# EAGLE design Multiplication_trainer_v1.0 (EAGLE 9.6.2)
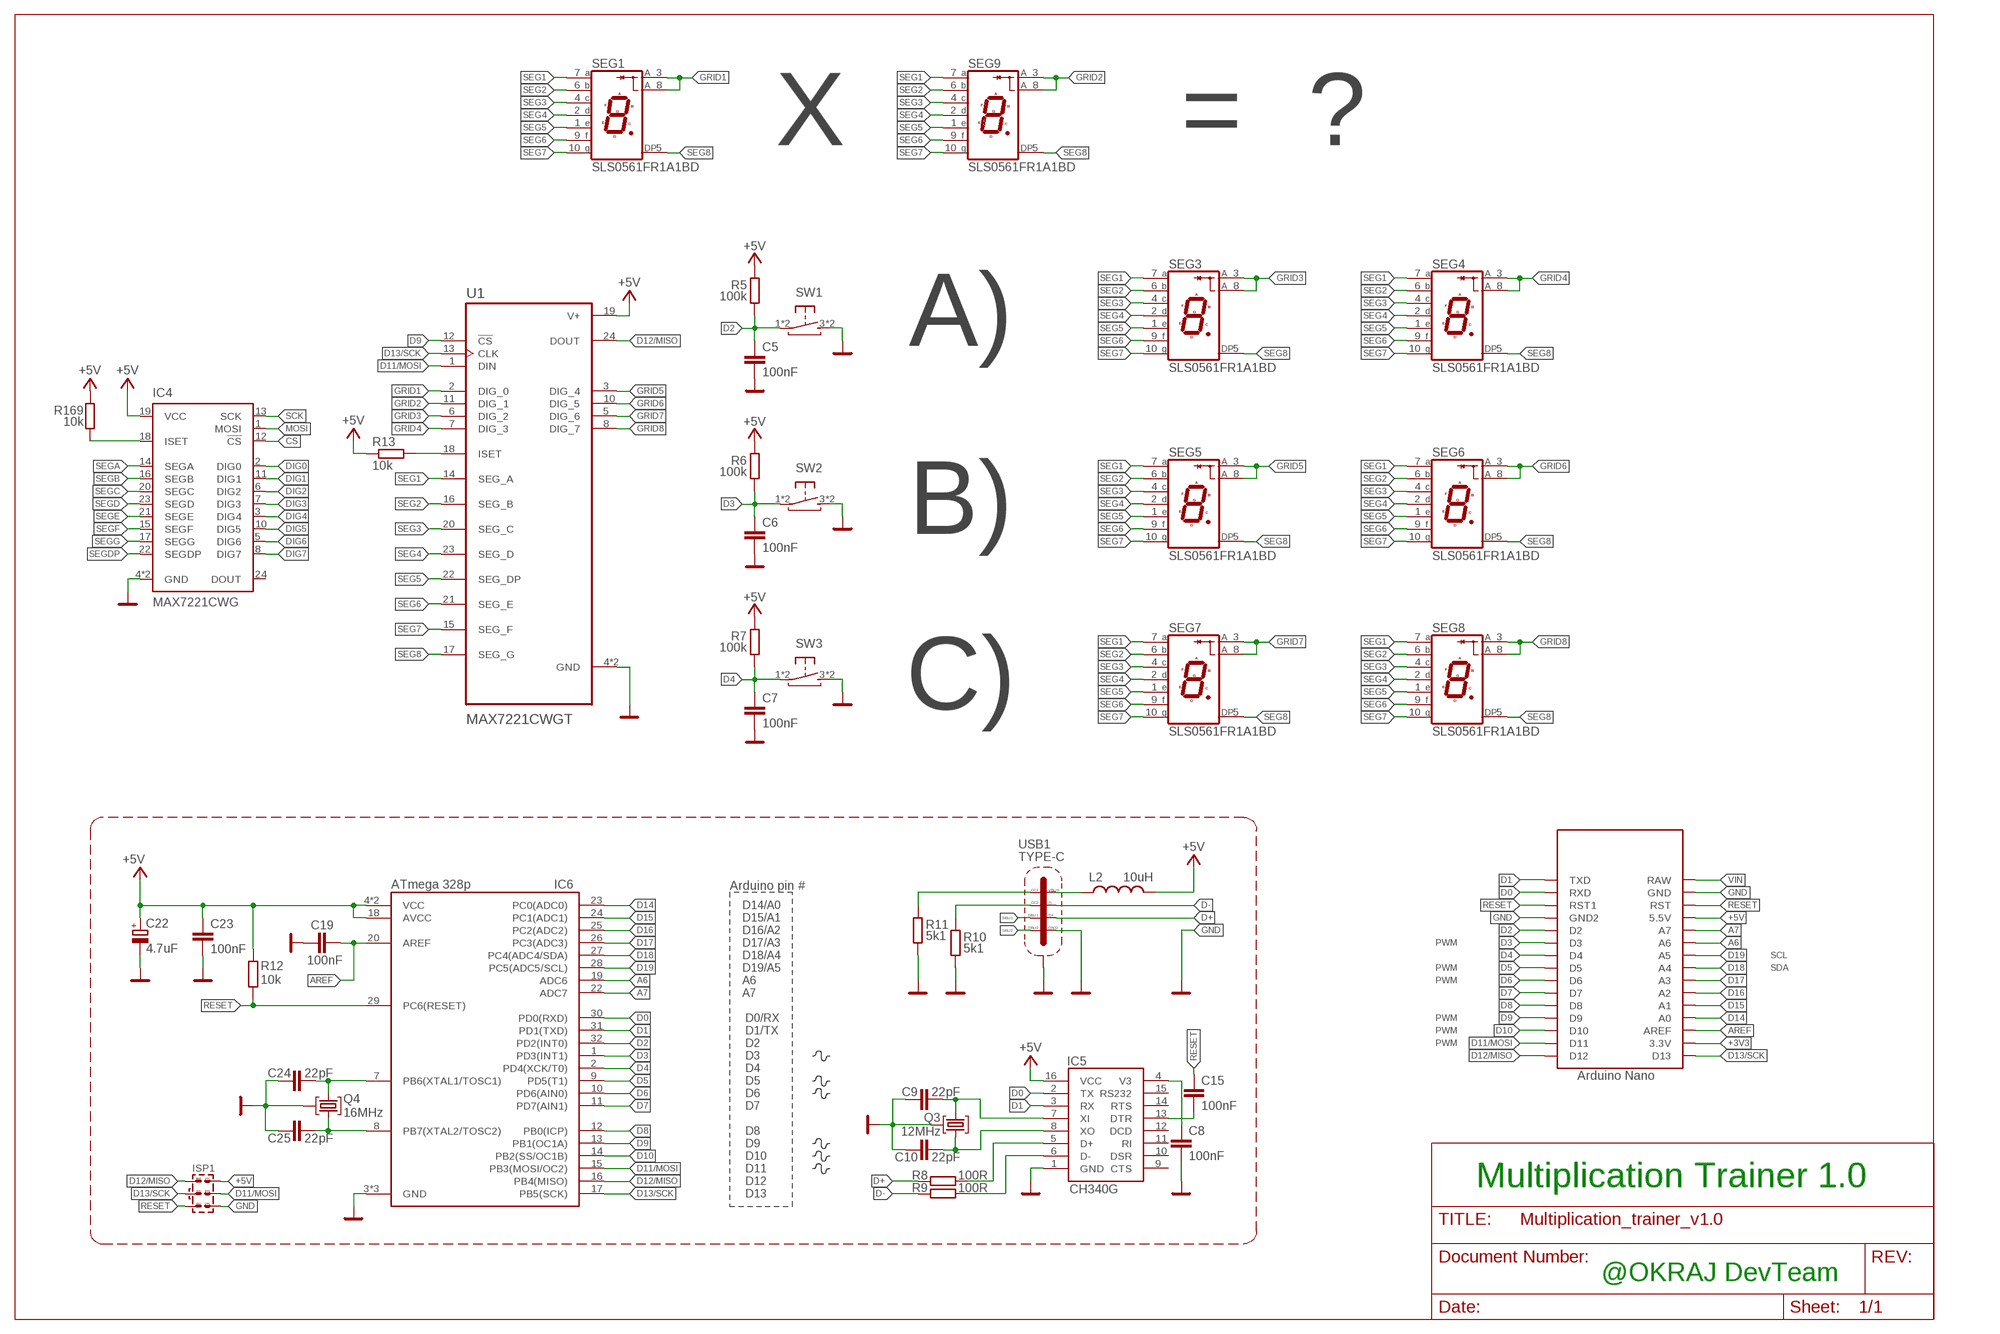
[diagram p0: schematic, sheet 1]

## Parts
C5  100nF  C-EUC0805  [C0805]
C6  100nF  C-EUC0805  [C0805]
C7  100nF  C-EUC0805  [C0805]
C8  100nF  C-EUC0603  [C0603]
C9  22pF  C-EUC0603  [C0603]
C10  22pF  C-EUC0603  [C0603]
C15  100nF  C-EUC0603  [C0603]
C19  100nF  C-EUC0603  [C0603]
C22  4.7uF  CPOL-EUSMCA  [SMC_A]
C23  100nF  C-EUC0603  [C0603]
C24  22pF  C-EUC0603  [C0603]
C25  22pF  C-EUC0603  [C0603]
IC4  MAX7221CWG  [SOIC127P1032X265-24N]
IC5  CH340G  CH340GSMD  [SOIC16]
IC6  ATmega 328p  ATMEGA328PQFP32N_ROUND-PADS  [QFP80P900X900X120-32N_ROUND-PADS]
ISP1  AVR-ISP-SPI  [AVR-ISP-SPI]
L2  10uH  L-USL0805  [R0805]
Q3  12MHz  KRYSTAL  [ILCX13-FF5F18-16.0000]
Q4  16MHz  KRYSTAL  [ILCX13-FF5F18-16.0000]
R5  100k  R-EU_R0805  [R0805]
R6  100k  R-EU_R0805  [R0805]
R7  100k  R-EU_R0805  [R0805]
R8  100R  R-EU_R0603  [R0603]
R9  100R  R-EU_R0603  [R0603]
R10  5k1  R-EU_R0603  [R0603]
R11  5k1  R-EU_R0603  [R0603]
R12  10k  R-EU_R0603  [R0603]
R13  10k  R-EU_R0805  [R0805]
R169  10k  R-EU_R0805  [R0805]
SEG1  SLS0561FR1A1BD  [SLS0561FR1A1BD]
SEG3  SLS0561FR1A1BD  [SLS0561FR1A1BD]
SEG4  SLS0561FR1A1BD  [SLS0561FR1A1BD]
SEG5  SLS0561FR1A1BD  [SLS0561FR1A1BD]
SEG6  SLS0561FR1A1BD  [SLS0561FR1A1BD]
SEG7  SLS0561FR1A1BD  [SLS0561FR1A1BD]
SEG8  SLS0561FR1A1BD  [SLS0561FR1A1BD]
SEG9  SLS0561FR1A1BD  [SLS0561FR1A1BD]
SW1  TACT-SW_BTNSMTJLC_6X6X4.5  [TACTSW_6X6X4.5_SMT]
SW2  TACT-SW_BTNSMTJLC_6X6X4.5  [TACTSW_6X6X4.5_SMT]
SW3  TACT-SW_BTNSMTJLC_6X6X4.5  [TACTSW_6X6X4.5_SMT]
U1  MAX7221CWGT  [SOIC127P1032X265-24N]
U$2  NANOTHT-NOUSB  [NANO-NOUSB]
USB1  TYPE-C  TYPE-C-31-M-12TYPE-C-31_L8.94_W7.3  [TYPE-C-31_L8.94_W7.3]

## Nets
+3V3: U$2.3.3V
+5V: C22.+ C23.1 IC4.19(VCC) IC5.16(VCC) IC6.4(VCC) IC6.6(VCC) IC6.18(AVCC) ISP1.2 L2.2 R5.1 R6.1 R7.1 R12.1 R13.1 R169.2 U1.19(V+) U$2.5V(5.5V)
A6: IC6.19(ADC6) U$2.A6
A7: IC6.22(ADC7) U$2.A7
AREF: C19.1 IC6.20(AREF) U$2.AREF
CS: IC4.12(!CS)
D0: IC5.2(TX) IC6.30(PD0(RXD)) U$2.RX1(RXD)
D1: IC5.3(RX) IC6.31(PD1(TXD)) U$2.TX0(TXD)
D2: C5.1 IC6.32(PD2(INT0)) R5.2 SW1.1(P) SW1.2(P) U$2.D2
D3: C6.1 IC6.1(PD3(INT1)) R6.2 SW2.1(P) SW2.2(P) U$2.D3
D4: C7.1 IC6.2(PD4(XCK/T0)) R7.2 SW3.1(P) SW3.2(P) U$2.D4
D5: IC6.9(PD5(T1)) U$2.D5
D6: IC6.10(PD6(AIN0)) U$2.D6
D7: IC6.11(PD7(AIN1)) U$2.D7
D8: IC6.12(PB0(ICP)) U$2.D8
D9: IC6.13(PB1(OC1A)) U1.12(!CS) U$2.D9
D10: IC6.14(PB2(SS/OC1B)) U$2.D10
D11/MOSI: IC6.15(PB3(MOSI/OC2)) ISP1.4 U1.1(DIN) U$2.D11
D12/MISO: IC6.16(PB4(MISO)) ISP1.1 U1.24(DOUT) U$2.D12
D13/SCK: IC6.17(PB5(SCK)) ISP1.3 U1.13(CLK) U$2.D13
D14: IC6.23(PC0(ADC0)) U$2.A0
D15: IC6.24(PC1(ADC1)) U$2.A1
D16: IC6.25(PC2(ADC2)) U$2.A2
D17: IC6.26(PC3(ADC3)) U$2.A3
D18: IC6.27(PC4(ADC4/SDA)) U$2.A4
D19: IC6.28(PC5(ADC5/SCL)) U$2.A5
D+: R8.1 USB1.A6(D+) USB1.B6(D+)
D-: R9.1 USB1.A7(D-) USB1.B7(D-)
DIG0: IC4.2(DIG0)
DIG1: IC4.11(DIG1)
DIG2: IC4.6(DIG2)
DIG3: IC4.7(DIG3)
DIG4: IC4.3(DIG4)
DIG5: IC4.10(DIG5)
DIG6: IC4.5(DIG6)
DIG7: IC4.8(DIG7)
GND: C5.2 C6.2 C7.2 C8.2 C9.2 C10.2 C19.2 C22.- C23.2 C24.2 C25.2 IC4.4(GND) IC4.9(GND) IC5.1(GND) IC6.3(GND) IC6.5(GND) IC6.21(GND) ISP1.6 Q3.P$2(GND) Q3.P$4(GND) Q4.P$2(GND) Q4.P$4(GND) R10.1 R11.1 SW1.3(S) SW1.4(S) SW2.3(S) SW2.4(S) SW3.3(S) SW3.4(S) U1.4(GND) U1.9(GND) U$2.GND U$2.GND1(GND2) USB1.A1/B12(GND) USB1.B1/A12(GND) USB1.SHIELD1(SHIELD) USB1.SHIELD2(SHIELD) USB1.SHIELD3(SHIELD) USB1.SHIELD4(SHIELD) USB1.SHIELD5(SHIELD) USB1.SHIELD6(SHIELD) USB1.SHIELD7(SHIELD) USB1.SHIELD8(SHIELD)
GRID1: SEG1.3(CA1) SEG1.8(CA2) U1.2(DIG_0)
GRID2: SEG9.3(CA1) SEG9.8(CA2) U1.11(DIG_1)
GRID3: SEG3.3(CA1) SEG3.8(CA2) U1.6(DIG_2)
GRID4: SEG4.3(CA1) SEG4.8(CA2) U1.7(DIG_3)
GRID5: SEG5.3(CA1) SEG5.8(CA2) U1.3(DIG_4)
GRID6: SEG6.3(CA1) SEG6.8(CA2) U1.10(DIG_5)
GRID7: SEG7.3(CA1) SEG7.8(CA2) U1.5(DIG_6)
GRID8: SEG8.3(CA1) SEG8.8(CA2) U1.8(DIG_7)
MOSI: IC4.1(MOSI)
N$1: C8.1 IC5.4(V3)
N$2: C9.1 IC5.7(XI) Q3.P$1
N$3: C10.1 IC5.8(XO) Q3.P$3
N$4: C15.2 IC5.13(DTR)
N$5: IC5.5(D+) R8.2
N$8: IC5.6(D-) R9.2
N$9: L2.1 USB1.A4/B9(VBUS) USB1.B4/A9(VBUS)
N$10: R10.2 USB1.B5(CC2)
N$11: R11.2 USB1.A5(CC1)
N$12: C24.1 IC6.7(PB6(XTAL1/TOSC1)) Q4.P$1
N$13: C25.1 IC6.8(PB7(XTAL2/TOSC2)) Q4.P$3
N$14: R13.2 U1.18(ISET)
N$131: IC4.18(ISET) R169.1
RESET: C15.1 IC6.29(PC6(RESET)) ISP1.5 R12.2 U$2.RST U$2.RST1
SBU1: USB1.A8(SBU1)
SBU2: USB1.B8(SBU2)
SCK: IC4.13(SCK)
SEG1: SEG1.7(A) SEG3.7(A) SEG4.7(A) SEG5.7(A) SEG6.7(A) SEG7.7(A) SEG8.7(A) SEG9.7(A) U1.14(SEG_A)
SEG2: SEG1.6(B) SEG3.6(B) SEG4.6(B) SEG5.6(B) SEG6.6(B) SEG7.6(B) SEG8.6(B) SEG9.6(B) U1.16(SEG_B)
SEG3: SEG1.4(C) SEG3.4(C) SEG4.4(C) SEG5.4(C) SEG6.4(C) SEG7.4(C) SEG8.4(C) SEG9.4(C) U1.20(SEG_C)
SEG4: SEG1.2(D) SEG3.2(D) SEG4.2(D) SEG5.2(D) SEG6.2(D) SEG7.2(D) SEG8.2(D) SEG9.2(D) U1.23(SEG_D)
SEG5: SEG1.1(E) SEG3.1(E) SEG4.1(E) SEG5.1(E) SEG6.1(E) SEG7.1(E) SEG8.1(E) SEG9.1(E) U1.22(SEG_DP)
SEG6: SEG1.9(F) SEG3.9(F) SEG4.9(F) SEG5.9(F) SEG6.9(F) SEG7.9(F) SEG8.9(F) SEG9.9(F) U1.21(SEG_E)
SEG7: SEG1.10(G) SEG3.10(G) SEG4.10(G) SEG5.10(G) SEG6.10(G) SEG7.10(G) SEG8.10(G) SEG9.10(G) U1.15(SEG_F)
SEG8: SEG1.5(DP) SEG3.5(DP) SEG4.5(DP) SEG5.5(DP) SEG6.5(DP) SEG7.5(DP) SEG8.5(DP) SEG9.5(DP) U1.17(SEG_G)
SEGA: IC4.14(SEGA)
SEGB: IC4.16(SEGB)
SEGC: IC4.20(SEGC)
SEGD: IC4.23(SEGD)
SEGDP: IC4.22(SEGDP)
SEGE: IC4.21(SEGE)
SEGF: IC4.15(SEGF)
SEGG: IC4.17(SEGG)
VIN: U$2.RAW
Unconnected: IC4.24(DOUT) IC5.9(CTS) IC5.10(DSR) IC5.11(RI) IC5.12(DCD) IC5.14(RTS) IC5.15(RS232)

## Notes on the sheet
- X | = | ?
- A)
- B)
- C)
- Arduino pin #
- D14/A0
- D15/A1
- D16/A2
- D17/A3 | PWM
- D18/A4 | SCL
- D19/A5 | PWM | SDA
- A6 | PWM
- A7
- D0/RX | PWM
- D1/TX | PWM
- D2 | PWM
- D3
- D4
- D5
- D6
- D7
- D8
- D9
- D10
- D11
- D12
- Multiplication Trainer 1.0
- D13
- @OKRAJ DevTeam

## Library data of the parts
C5-C7 = rcl:C-EU: CAPACITOR, European symbol
C8 C15 C19 C23 = rcl:C-EU: CAPACITOR, European symbol; LCSC_PART: C49678; SPICEPREFIX: C
C9 C10 C24 C25 = rcl:C-EU: CAPACITOR, European symbol; LCSC_PART: C1804; SPICEPREFIX: C
C22 = rcl:CPOL-EU: POLARIZED CAPACITOR, European symbol; LCSC_PART: C111040; ROT: 180; SPICEPREFIX: C
IC4 = MAX7221:MAX7221CWG: 7 SEGMENT 8 DIGIT DRIVER 24SOIC Datasheet; MOUSER_NO: 710-157119S12701
IC5 = ch340g:CH340G; LCSC_PART: C14267
IC6 = ATMEGA328P-ANR:ATMEGA328P: 8-bit Microcontrollers - MCU AVR 32K FLSH 2K SRAM 1KB EE-20 MHZ 105C Source: Datasheet; LCSC_PART: C14877; ROT: 270
ISP1 = #Ondra2:AVR-ISP-SPI
L2 = rcl:L-US: INDUCTOR, American symbol; LCSC_PART: C281113
Q3 = #Marek:KRYSTAL: Monolithic Crystal Filters Source: www.vanlong.com; LCSC_PART: C9002
Q4 = #Marek:KRYSTAL: Monolithic Crystal Filters Source: www.vanlong.com; LCSC_PART: C13738
R5-R7 = resistor:R-EU_: RESISTOR, European symbol
R8 R9 R12 R13 R169 = rcl:R-EU_: RESISTOR, European symbol; SPICEPREFIX: R
R10 R11 = rcl:R-EU_: RESISTOR, European symbol; LCSC_PART: C27834; SPICEPREFIX: R
SEG1 SEG3-SEG9 = #my:SLS0561FR1A1BD; LCSC_PART: C226002
SW1-SW3 = #Ondra2:TACT-SW_BTN; LCSC_PART: C127509
U1 = MAX7221CWGT:MAX7221CWGT: Check availability; AVAILABILITY: In Stock; DESCRIPTION: IC DRVR 7 SEGMNT 8 DIGIT 24SOIC; MF: Maxim Integrated; MP: MAX7221CWG+T; PACKAGE: SOIC-24 Maxim; PRICE: None; PURCHASE-URL: https://pricing.snapeda.com/search/part/MAX7221CWG+T/?ref=eda
U$2 = Arduino-clone:NANO: Arduino Nano
USB1 = #Marek:TYPE-C-31-M-12; LCSC_PART: C165948; ROT: 180

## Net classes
0 default: width 0.127 mm, drill 0.2 mm, clearance 0.127 mm

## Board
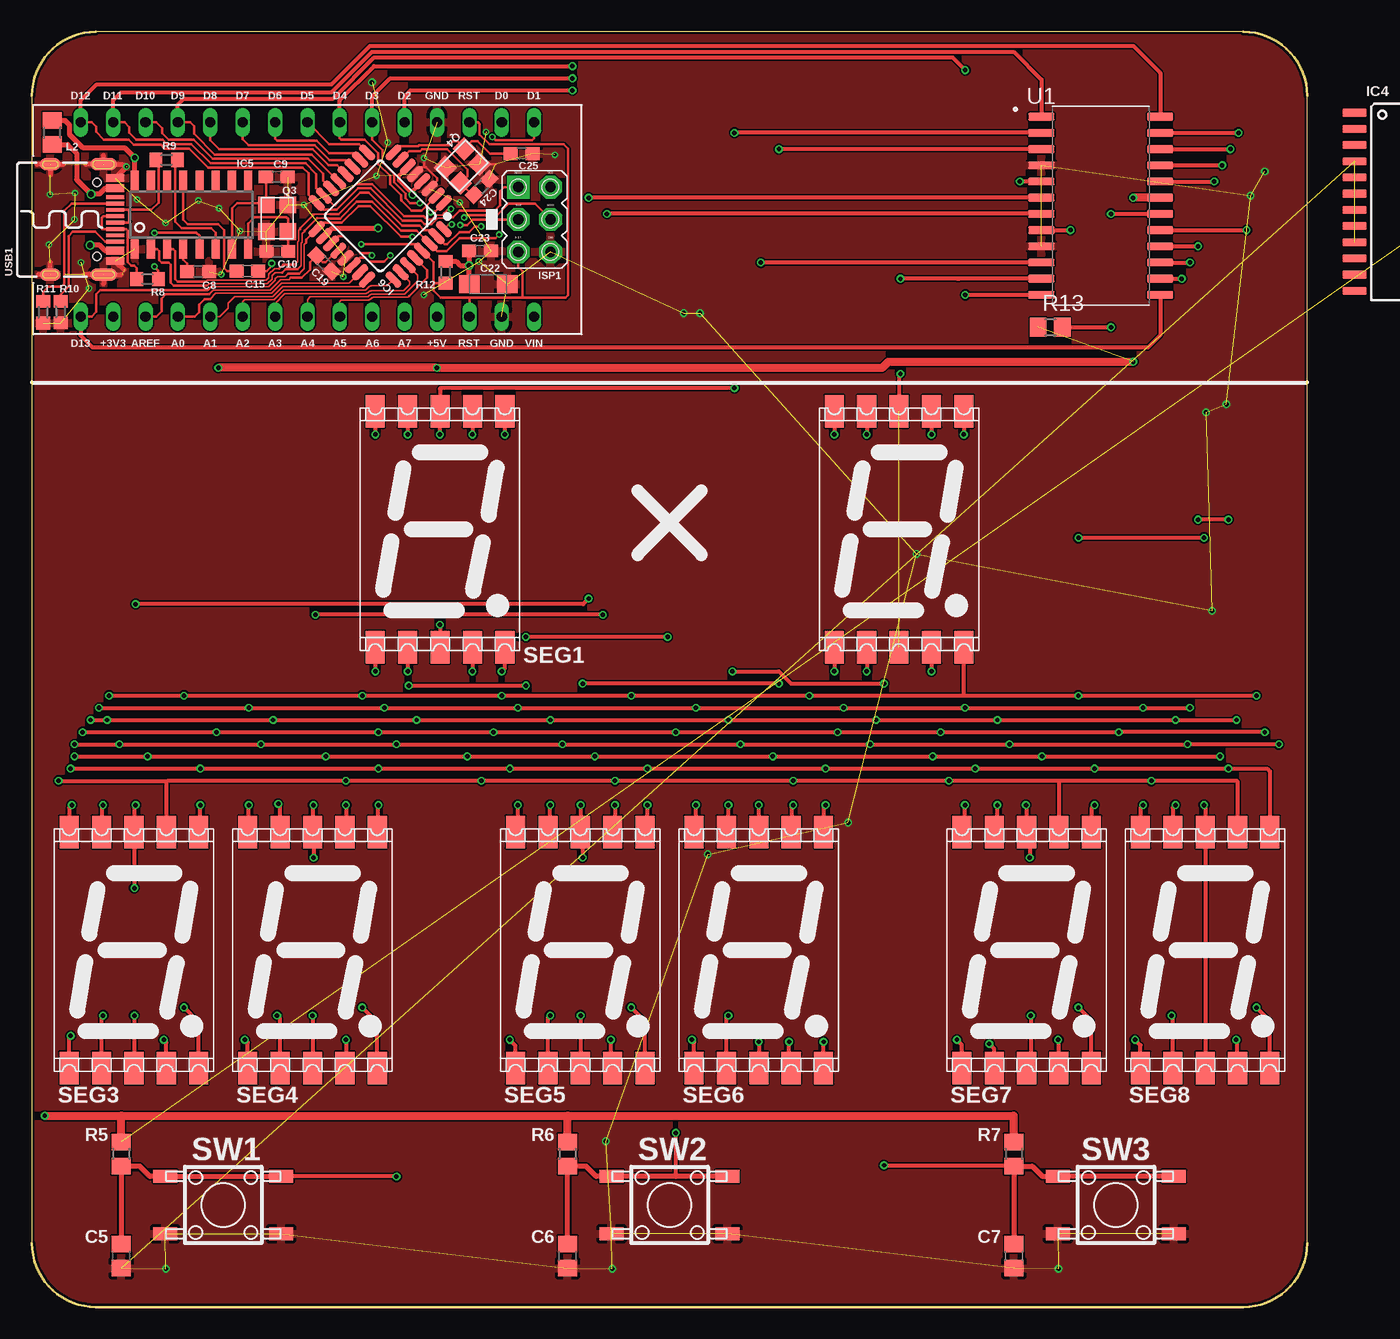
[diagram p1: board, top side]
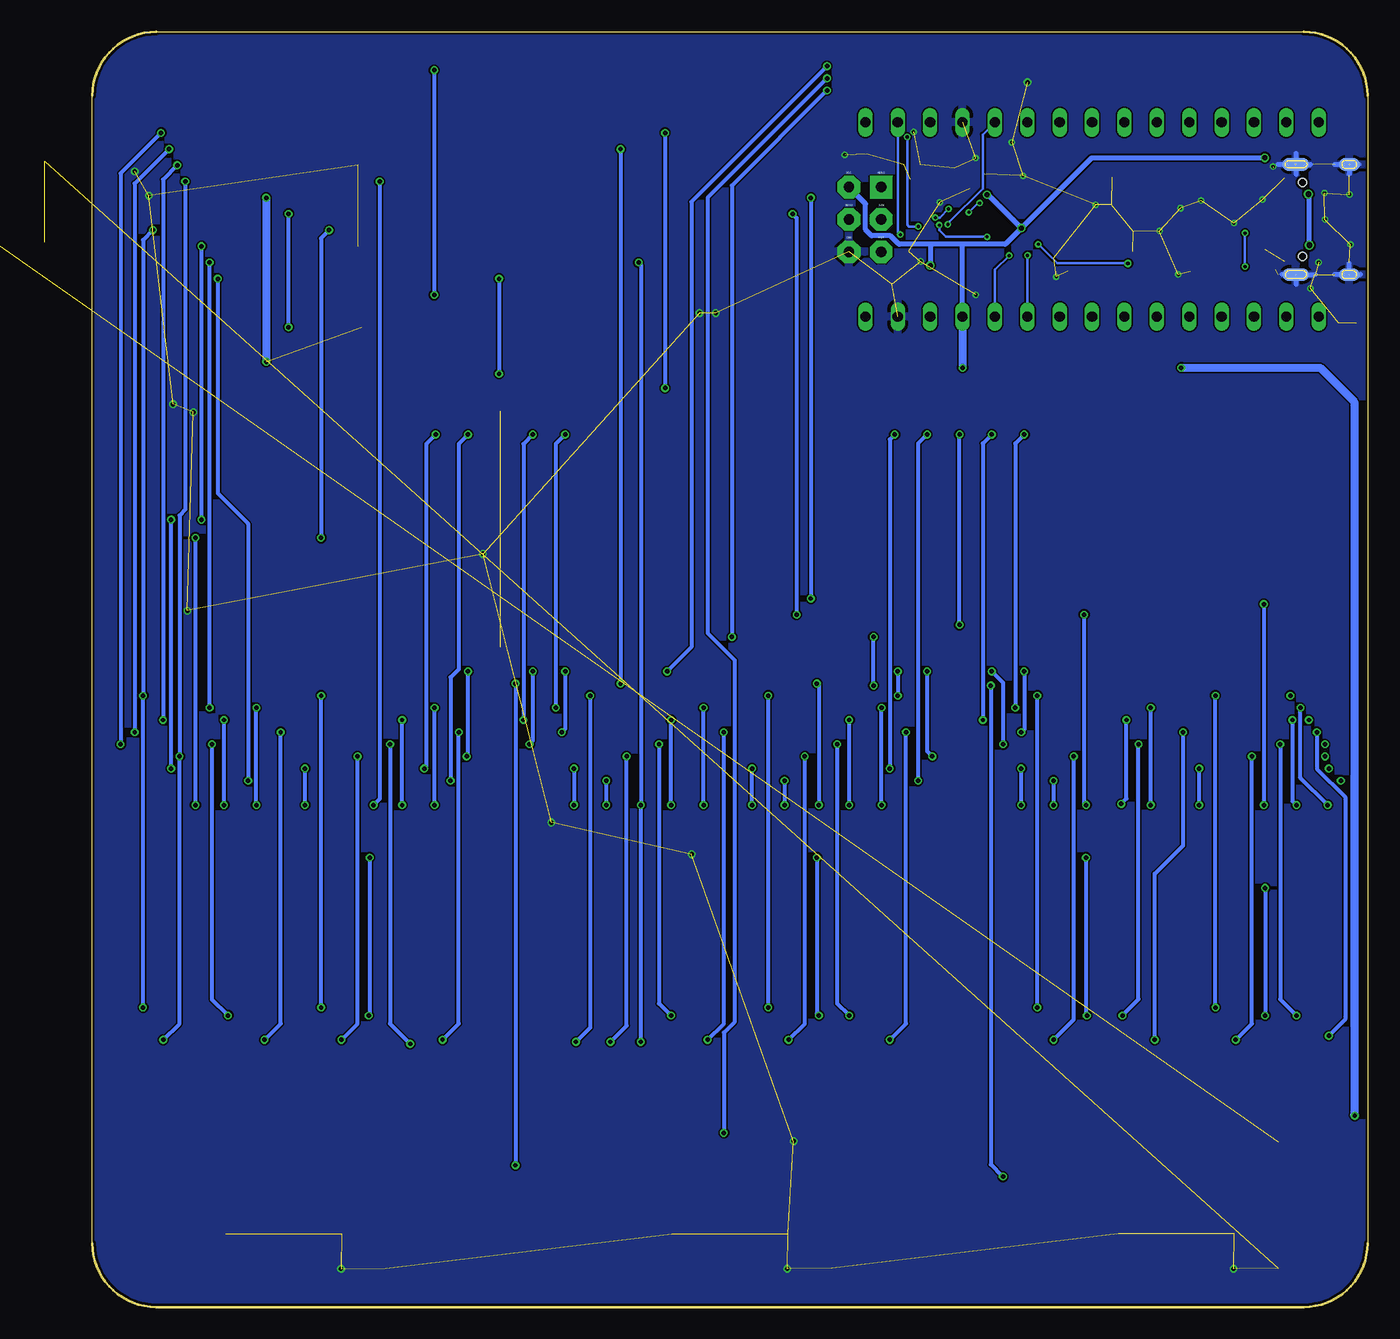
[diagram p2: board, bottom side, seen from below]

Size 100 x 100 mm. Coordinates in mm from the lower left corner, seen from the top.
Outline: 100,5 100,95 arc90 95,100 5,100 arc90 0,95 0,5 arc90 5,0 95,0 arc90 100,5
Copper layers (1*16): Top 0.035mm / dielectric 1.6mm / Bottom 0.035mm
Design rules "jlcpcb-2layers_od-Ondry3-assembly-tight": minimum track width 5mil, minimum drill 0.2mm, track to track 5mil, track to pad 5mil, pad to pad 5mil, via to via 5mil, smd to smd 5mil, copper to edge 0.2mm, drill to drill 6mil, minimum pad ring 0.13mm, minimum via ring 0.13mm, stop-mask expansion 4mil, vias tented up to drill 0.6mm, thermal gap 10mil

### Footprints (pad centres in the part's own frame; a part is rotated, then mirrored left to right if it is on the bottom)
C0805 = smd 1.3 x 1.5: 1 -0.95,0; 2 0.95,0
C0603 = smd 1.1 x 1: 1 -0.85,0; 2 0.85,0
SMC_A = smd 1.6 x 1.4: + -1.5,0; - 1.5,0
SOIC127P1032X265-24N = smd 1.925 x 0.65: 1 -4.712,6.985; 2 -4.712,5.715; 3 -4.712,4.445; 4 -4.712,3.175; 5 -4.712,1.905; 6 -4.712,0.635; 7 -4.712,-0.635; 8 -4.712,-1.905; 9 -4.712,-3.175; 10 -4.712,-4.445; 11 -4.712,-5.715; 12 -4.712,-6.985; 13 4.712,-6.985; 14 4.712,-5.715; 15 4.712,-4.445; 16 4.712,-3.175; 17 4.712,-1.905; 18 4.712,-0.635; 19 4.712,0.635; 20 4.712,1.905; 21 4.712,3.175; 22 4.712,4.445; 23 4.712,5.715; 24 4.712,6.985
SOIC16 = smd 0.635 x 1.524: 1 -4.445,-2.695; 2 -3.175,-2.695; 3 -1.905,-2.695; 4 -0.635,-2.695; 5 0.635,-2.695; 6 1.905,-2.695; 7 3.175,-2.695; 8 4.445,-2.695; 9 4.445,2.695; 10 3.175,2.695; 11 1.905,2.695; 12 0.635,2.695; 13 -0.635,2.695; 14 -1.905,2.695; 15 -3.175,2.695; 16 -4.445,2.695
QFP80P900X900X120-32N_ROUND-PADS = smd 1.499 x 0.584: 1 -4.25,2.8; 2 -4.25,2; 3 -4.25,1.2; 4 -4.25,0.4; 5 -4.25,-0.4; 6 -4.25,-1.2; 7 -4.25,-2; 8 -4.25,-2.8; 17 4.25,-2.8; 18 4.25,-2; 19 4.25,-1.2; 20 4.25,-0.4; 21 4.25,0.4; 22 4.25,1.2; 23 4.25,2; 24 4.25,2.8 | smd 0.584 x 1.499: 9 -2.8,-4.25; 10 -2,-4.25; 11 -1.2,-4.25; 12 -0.4,-4.25; 13 0.4,-4.25; 14 1.2,-4.25; 15 2,-4.25; 16 2.8,-4.25; 25 2.8,4.25; 26 2,4.25; 27 1.2,4.25; 28 0.4,4.25; 29 -0.4,4.25; 30 -1.2,4.25; 31 -2,4.25; 32 -2.8,4.25
AVR-ISP-SPI = drill 0.813 pad 1.778 square: 1 -1.27,2.54 | drill 0.813 pad 1.778 octagon: 2 1.27,2.54; 3 -1.27,0; 4 1.27,0; 5 -1.27,-2.54; 6 1.27,-2.54
R0805 = smd 1.3 x 1.5: 1 -0.95,0; 2 0.95,0
ILCX13-FF5F18-16.0000 = smd 1.3 x 1.3: P$1 -1.05,-0.85; P$2 1.05,-0.85; P$3 1.05,0.85; P$4 -1.05,0.85
R0603 = smd 1 x 1.1: 1 -0.85,0; 2 0.85,0
SLS0561FR1A1BD = smd 1.5 x 2.54: 1 -5.08,-9.25; 2 -2.54,-9.25; 3 0,-9.25; 4 2.54,-9.25; 5 5.08,-9.25; 6 5.08,9.25; 7 2.54,9.25; 8 0,9.25; 9 -2.54,9.25; 10 -5.08,9.25
TACTSW_6X6X4.5_SMT = smd 1.9 x 1: 1 -4.55,2.25; 2 4.55,2.25; 3 -4.55,-2.25; 4 4.55,-2.25
SOIC127P1032X265-24N' = smd 2.05 x 0.59: 1 -4.655,6.985; 2 -4.655,5.715; 3 -4.655,4.445; 4 -4.655,3.175; 5 -4.655,1.905; 6 -4.655,0.635; 7 -4.655,-0.635; 8 -4.655,-1.905; 9 -4.655,-3.175; 10 -4.655,-4.445; 11 -4.655,-5.715; 12 -4.655,-6.985; 13 4.655,-6.985; 14 4.655,-5.715; 15 4.655,-4.445; 16 4.655,-3.175; 17 4.655,-1.905; 18 4.655,-0.635; 19 4.655,0.635; 20 4.655,1.905; 21 4.655,3.175; 22 4.655,4.445; 23 4.655,5.715; 24 4.655,6.985
NANO-NOUSB = drill 0.8 long: 3.3V -7.62,15.24; 5V -7.62,-10.16; A0 -7.62,10.16; A1 -7.62,7.62; A2 -7.62,5.08; A3 -7.62,2.54; A4 -7.62,0; A5 -7.62,-2.54; A6 -7.62,-5.08; A7 -7.62,-7.62; AREF -7.62,12.7; D2 7.62,-7.62; D3 7.62,-5.08; D4 7.62,-2.54; D5 7.62,0; D6 7.62,2.54; D7 7.62,5.08; D8 7.62,7.62; D9 7.62,10.16; D10 7.62,12.7; D11 7.62,15.24; D12 7.62,17.78; D13 -7.62,17.78; GND -7.62,-15.24; GND1 7.62,-10.16; RAW -7.62,-17.78; RST -7.62,-12.7; RST1 7.62,-12.7; RX1 7.62,-15.24; TX0 7.62,-17.78
TYPE-C-31_L8.94_W7.3 = smd 0.6 x 1.45: A1/B12 -3.25,3.885; A4/B9 -2.45,3.885; B1/A12 3.25,3.885; B4/A9 2.45,3.885 | smd 0.3 x 1.45: A5 -1.25,3.885; A6 -0.25,3.885; A7 0.25,3.885; A8 1.25,3.885; B5 1.75,3.885; B6 0.75,3.885; B7 -0.75,3.885; B8 -1.75,3.885 | smd 1 x 2.1: SHIELD1 -4.32,2.97; SHIELD2 4.32,2.97 | smd 1 x 1.6: SHIELD3 -4.32,-1.21; SHIELD4 4.32,-1.21 | smd 1 x 2.1 bottom: SHIELD5 -4.316,2.97; SHIELD8 4.316,2.97 | smd 1 x 1.6 bottom: SHIELD6 -4.316,-1.21; SHIELD7 4.316,-1.21 | hole 0.65: -2.89,2.44; 2.89,2.44

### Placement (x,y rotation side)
C5  7,4 270 top
C6  42,4 270 top
C7  77,4 270 top
C8  13.04,81.2 0 top
C9  19.19,88.62 0 top
C10  19.25,82.78 180 top
C15  16.89,81.24 180 top
C19  22.91,81.85 315 top
C22  35.79,80.23 0 top
C23  35.14,82.82 0 top
C24  35.26,87.83 45 top
C25  38.39,90.46 0 top
IC4  not placed on the board
IC5  12.51,85.66 0 top
IC6  27.31,85.56 225 top
ISP1  39.4,85.29 0 top
L2  1.59,92.11 90 top
Q3  19.22,85.38 270 top
Q4  33.75,89.49 45 top
R5  7,12 270 top
R6  42,12 270 top
R7  77,12 270 top
R8  9.06,80.62 0 top
R9  10.56,89.96 0 top
R10  2.24,78.02 90 top
R11  0.87,78.02 90 top
R12  32.44,81.15 270 top
R13  79.85,76.83 0 top
R169  not placed on the board
SEG1  32,61 0 top
SEG3  8,28 0 top
SEG4  22,28 0 top
SEG5  43,28 0 top
SEG6  57,28 0 top
SEG7  78,28 0 top
SEG8  92,28 0 top
SEG9  68,61 0 top
SW1  15,8 0 top
SW2  50,8 0 top
SW3  85,8 0 top
U1  MAX7221CWGT  [SOIC127P1032X265-24N']  83.82,86.36 0 top
U$2  21.6,85.29 90 top
USB1  2.64,85.29 270 top

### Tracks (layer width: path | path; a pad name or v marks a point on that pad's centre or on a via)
+5V  (via drill 0.35, 0.35 pad 0.55, 0.4)  (3 unrouted)
  Top 0.305: IC6.4 29.84,87.52 | 29.85,87.52 29.84,87.52 | 29.84,87.52 29.62,87.52 28.78,88.36 28.78,88.73 IC6.6
  Top 0.406: L2.2 2.59,93.06 2.93,92.72 2.93,91.98 4.02,90.88 7.3,90.88 v8.06,90.13 IC5.16 | IC6.18 23.52,84.6 27.13,84.6 v27.15,84.61 | v29.85,87.24 29.85,87.52 | C22.+ v34.29,81.67 | v34.29,81.67 v34.29,81.68 | C23.1 v34.29,81.67 | v34.29,81.67 | R12.1 33.25,82 33.58,81.67 v34.29,81.67
  Top 0.61: R5.1 7,15 | R6.1 42,15 | R7.1 77,15 42,15 | v1,15 7,15 | 7,15 42,15 | v14.61,73.66 v31.75,73.66 66.67,73.66 67.15,74.14 v86.36,74.14 | U1.19 v86.36,87
  Bottom 0.406: v27.15,84.61 29.77,87.24 v29.85,87.24 | v27.15,84.61 28.42,83.34 31.75,83.34 | v34.29,81.68 34.29,83.26 34.21,83.34 | 31.75,83.34 34.21,83.34 | 34.21,83.34 36.74,83.34 37.42,84.02 38.89,84.02 39.37,84.5 39.37,86.53 ISP1.2 | v27.15,84.61 21.63,90.13 v8.06,90.13 | U$2.5V 31.76,83.33 31.75,83.34
  Bottom 0.61: v14.61,73.66 3.71,73.66 1.05,71 1.05,15.05 v1,15 | U$2.5V v31.76,73.67 v31.75,73.66 | v86.36,87 v86.36,74.14
A6  (via drill 0.25)
  Top 0.203: IC6.19 24.02,83.96 24.39,83.96 25.72,82.63 26.51,82.63 v26.67,82.47
  Bottom 0.203: U$2.A6 v26.68,82.47 v26.67,82.47
A7  (via drill 0.25)
  Top 0.203: IC6.22 25.75,82.3 26.13,82.3 26.44,81.98 27.61,81.98 v28.09,82.46 v28.1,82.46
  Bottom 0.203: U$2.A7 29.22,81.34 v28.1,82.46
AREF
  Top 0.127: 13.89,79.42 14.22,79.75 18.67,79.75 19.49,80.57 20.16,80.57 20.3,80.71
  Top 0.203: U$2.AREF 9.72,77.67 10.16,78.1 10.16,79.09 10.49,79.42 13.89,79.42 | 20.3,80.71 21.16,80.71 21.8,81.34 21.8,81.94 C19.1 22.81,81.95 23.02,81.95 23.91,82.84 IC6.20
D0  (via drill 0.25)
  Top 0.127: 22.35,85.4 23.2,85.4 23.24,85.36 | 13.65,80.08 13.73,80.08 13.91,80.26 18.46,80.26 18.82,80.62 18.82,80.88 19.08,81.14 19.63,81.14 | 20.82,81.39 21.09,81.66 21.09,83.42 21.17,83.5 21.17,84.17 21.37,84.37
  Top 0.203: 13.65,80.08 11.11,80.08 10.87,80.32 10.87,81.76 10.72,81.92 10.16,81.92 9.97,82.11 9.97,82.8 9.81,82.96 IC5.2 | v36.63,84.1 36.35,83.81 33.55,83.81 32.53,82.79 31.79,82.79 IC6.30 30.16,84.42 28.93,84.42 26.67,86.68 25.47,86.68 24.15,85.36 23.24,85.36 | 22.35,85.4 21.37,84.41 21.37,84.37 | 19.63,81.14 19.89,81.39 20.82,81.39
  Bottom 0.203: v36.63,84.1 36.83,84.3 36.83,92.9 U$2.RX1
D1  (via drill 0.25)
  Top 0.127: 22.03,85.68 22.07,85.72 23.36,85.72 23.37,85.72 | 13.57,80.41 13.65,80.41 13.75,80.51 18.36,80.51 18.57,80.73 18.57,80.98 19.02,81.43 19.38,81.43 | 20.62,81.74 20.84,81.96 20.84,83.53 20.91,83.61 20.91,84.43 21.03,84.54
  Top 0.203: 21.03,84.54 21.03,84.62 22.09,85.68 22.03,85.68 | 23.37,85.72 24.03,85.72 25.72,87.41 26.41,87.41 29.01,84.81 30.38,84.81 30.72,84.47 31.24,84.47 IC6.31 32.37,83.34 32.57,83.34 33.53,84.3 34.27,84.3 34.71,84.74 v35.23,84.74 | v36.1,91.76 36.34,91.52 39.22,91.52 39.38,91.68 U$2.TX0 | 20.62,81.74 19.69,81.74 19.38,81.43 | IC5.3 11.08,82.96 11.24,82.8 11.24,80.62 11.44,80.41 13.57,80.41
  Bottom 0.203: v35.23,84.74 35.95,84.74 36.1,84.89 v36.1,91.76
D2  (via drill 0.25, 0.35)
  Top 0.203: IC6.32 32.66,84.9 32.91,84.9 v32.92,84.91
  Top 0.305: U$2.D2 29.22,94.94 29.69,95.41 v42.39,95.41 | v28.59,10.23 28.57,10.25 SW1.2 | v49.85,52.55 v38.73,52.55 | v29.54,48.74 v38.73,48.74
  Top 0.406: SW1.2 SW1.1 9.25,10.25 8.45,11.05 R5.2 C5.1
  Bottom 0.203: v32.92,84.91 32.78,85.04 32.78,85.1 30.17,87.7 30.17,91.95 U$2.D2
  Bottom 0.305: v42.39,95.41 49.85,87.95 v49.85,52.55 | v38.73,48.74 v38.73,52.55 | v29.54,48.74 29.54,11.18 v28.59,10.23
D3  (via drill 0.25, 0.35)
  Top 0.127: 27.55,89.7 27.46,89.79 27.46,90.45 27.51,90.5
  Top 0.203: IC6.1 31.64,85.93 31.34,85.93 v31.26,85.85 | v30.41,86.58 29.66,86.58 29.29,86.94 29.29,87.31 28.4,88.21 28.4,88.86 27.55,89.7 | 27.51,90.5 27.51,90.72 26.68,91.56 U$2.D3
  Top 0.305: U$2.D3 26.68,94.94 28.1,96.36 v42.39,96.36 | v50.48,13.65 50.48,10.25
  Top 0.406: C6.1 R6.2 43.45,11.05 44.25,10.25 SW2.1 50.48,10.25 SW2.2
  Bottom 0.203: v31.26,85.85 30.54,86.58 v30.41,86.58
  Bottom 0.305: v50.48,13.65 50.48,21.51 49.62,22.37 49.62,50.71 51.75,52.84 51.75,87 v42.39,96.36
D4  (via drill 0.35)
  Top 0.203: U$2.D4 24.14,91.67 24.25,91.56 26.07,91.56 27.16,90.48 27.16,89.63 28.07,88.72 28.07,88.07 28.96,87.18 28.96,86.81 28.97,86.8 28.97,86.76 29.77,85.96 30.54,85.96 IC6.2
  Top 0.305: U$2.D4 24.14,94.62 26.83,97.31 v42.39,97.31 | v66.82,11.11 76.94,11.11 R7.2 | v54.93,49.85 58.58,49.85 59.53,48.9 v66.82,48.9
  Top 0.406: SW3.2 SW3.1 79.25,10.25 78.45,11.05 R7.2 C7.1
  Bottom 0.305: v66.82,48.9 v66.82,11.11 | v54.93,49.85 53.02,51.75 53.02,86.68 v42.39,97.31
D5
  Top 0.203: IC6.9 25.64,91.2 23.3,91.2 U$2.D5
D6
  Top 0.203: IC6.10 25.21,90.5 23.29,90.5 22.31,91.48 19.22,91.48 19.06,91.64 U$2.D6
D7
  Top 0.203: IC6.11 25.11,89.42 24.6,89.93 23.34,89.93 22.16,91.12 16.99,91.12 16.52,91.59 U$2.D7
D8
  Top 0.203: U$2.D8 13.98,91.5 14.68,90.79 22.02,90.79 23.28,89.53 23.92,89.53 IC6.12
D9  (via drill 0.35)
  Top 0.203: U$2.D9 12.42,92.91 12.7,92.62 12.7,92.02 14.33,90.38 21.93,90.38 IC6.13
  Top 0.305: U$2.D9 11.44,94.31 11.91,94.77 23.63,94.77 26.85,97.99 72.19,97.99 v73.18,97 | v73.18,79.38 U1.12
  Bottom 0.305: v73.18,97 v73.18,79.38
D10
  Top 0.203: IC6.14 22.84,88.34 22.84,88.86 21.67,90.04 14.17,90.04 12.67,91.54 10.71,91.54 10.2,92.06 10.2,92.43 9.72,92.91 U$2.D10
  Top 0.305: U$2.D10
D11/MOSI  (via drill 0.25)
  Top 0.127: 32.31,85.77 32.18,85.64 31.68,85.64 31.32,85.28 31.29,85.28
  Top 0.203: U$2.D11 7.25,92.91 7.63,92.53 7.63,92.08 8.18,91.53 10.26,91.53 10.58,91.21 12.48,91.21 14,89.69 21.45,89.69 22.3,88.84 22.3,87.75 IC6.15 23.66,86.39 23.76,86.39 25.43,88.06 26.68,88.06 29.18,85.57 30.72,85.57 31.01,85.28 31.29,85.28 | v32.86,86.12 32.66,86.12 32.31,85.77 | v33.89,85.44 34.07,85.62 36.48,85.62 37.39,86.52 39.44,86.52 ISP1.4
  Top 0.305: U$2.D11 6.36,94.62 6.99,95.25 23.5,95.25 26.67,98.42 76.99,98.42 79.17,96.25 U1.1
  Bottom 0.203: v32.86,86.12 33.55,85.44 v33.89,85.44
D12/MISO
  Top 0.127: 31.35,84.93 31.8,85.38 32.38,85.38
  Top 0.203: U$2.D12 4.67,92.91 5.02,92.56 5.02,92.16 5.64,91.53 7.6,91.53 7.97,91.16 10.12,91.16 10.42,90.86 12.32,90.86 13.82,89.35 21.24,89.35 21.69,88.9 21.69,87.23 IC6.16 22.87,86.05 23.9,86.05 25.58,87.73 26.55,87.73 29.08,85.2 30.53,85.2 30.8,84.93 31.35,84.93 | ISP1.1 37.03,87.83 36.71,87.51 36.71,86.4 36.28,85.97 33.53,85.97 33.03,85.46 32.46,85.46 32.38,85.38
  Top 0.305: U$2.D12 3.82,94.62 5.08,95.89 23.5,95.89 26.51,98.9 86.36,98.9 88.47,96.79 U1.24
D13/SCK  (via drill 0.25)
  Top 0.127: 13.73,79.75 13.81,79.75 14.06,80 18.57,80 19.08,80.52 19.08,80.64 19.26,80.82 19.87,80.82 20.08,81.04 | 20.95,81.04 21.35,81.44 21.35,83.32 21.5,83.47
  Top 0.203: U$2.D13 4.67,77.67 5.05,78.05 5.05,79.43 5.37,79.75 13.73,79.75 | 21.5,83.47 21.5,83.71 IC6.17 22.82,85.03 24.29,85.03 25.61,86.35 26.53,86.35 28.95,83.93 v29.84,83.93 | v33.58,84.85 34.13,84.85 34.57,85.29 ISP1.3 | 20.08,81.04 20.95,81.04
  Top 0.305: U$2.D13 3.82,76.19 4.76,75.25 87.52,75.25 88.47,76.2 U1.13
  Bottom 0.203: v29.84,83.93 33.05,83.93 33.58,84.45 v33.58,84.85
D14
  Top 0.127: 13.97,79.06 14.41,79.5 18.78,79.5 19.57,80.29 24.86,80.29 IC6.23
  Top 0.203: U$2.A0 12.75,77.67 13.11,78.02 13.11,78.61 13.55,79.06 13.97,79.06
D15
  Top 0.127: U$2.A1 14.72,77.67 15.4,78.34 15.4,78.74 15.9,79.24 18.88,79.24 19.66,80.02 25.73,80.02 IC6.24
D16
  Top 0.127: U$2.A2 16.52,78.84 16.67,78.99 18.99,78.99 19.73,79.73 26.02,79.73 arc45 26.24,79.82 26.42,80 arc-45 26.64,80.09 27.85,80.09 IC6.25
D17
  Top 0.127: U$2.A3 19.06,78.7 19.83,79.47 26.12,79.47 arc45 26.35,79.57 26.38,79.6 arc-45 26.61,79.69 29.13,79.69 29.61,80.17 29.61,80.41 28.91,81.11 IC6.26
D18
  Top 0.127: U$2.A4 21.6,78.99 21.83,79.22 26.23,79.22 arc45 26.45,79.31 26.49,79.35 arc-45 26.71,79.44 29.24,79.44 30.24,80.44 30.24,80.94 IC6.27
D19
  Top 0.127: U$2.A5 24.14,78.86 24.25,78.97 26.33,78.97 arc45 26.56,79.06 26.59,79.09 arc-45 26.82,79.18 29.47,79.18 29.58,79.29
  Top 0.203: IC6.28 31,81.31 31,80.71 29.58,79.29
D+
  Top 0.203: USB1.A6 5.59,85.54 5.45,85.4 5.45,84.61 5.53,84.54 USB1.B6 7.38,84.54 7.51,84.4 7.51,81.94 7.78,81.68 8.02,81.68 8.21,81.48 R8.1
D-
  Top 0.203: USB1.A7 7.56,85.04 7.64,85.12 7.64,85.9 7.58,85.96 7.5,86.04 | 7.5,86.04 USB1.B7 | R9.1 9.92,89.75 9.92,86.6 9.36,86.04 7.5,86.04
GND  (via drill 0.25, 0.35)  (78 unrouted)
  Top 0.203: IC6.3 31.77,88.33 31.77,88.52 30.91,89.37 | 30.91,89.37 30.56,89.37 IC6.5 | 30.91,89.37 30.75,89.54 v30.75,90.1 | Q4.P$2 36.37,89.64
  Top 0.406: 1.43,81.9 USB1.SHIELD4 0.51,80.97 | USB1.SHIELD2 7.02,80.97 | USB1.SHIELD2 5.61,80.25 | USB1.SHIELD2 4.13,80.97 | USB1.SHIELD3 2.48,89.61 | USB1.SHIELD3 | USB1.SHIELD3 1.43,88.78 | USB1.SHIELD3 0.4,89.61 | USB1.B1/A12 7.22,81.34 | USB1.A1/B12 7.35,89.36 | 7.35,89.36 7.38,89.39 | USB1.SHIELD1 5.61,90.31 | USB1.SHIELD1 7.11,89.61 7.35,89.36 | USB1.SHIELD1 4.25,89.61
  Bottom 0.406: USB1.SHIELD6 1.43,88.82 | USB1.SHIELD6 0.66,89.6 | USB1.SHIELD6 2.58,89.6 | USB1.SHIELD5 4.48,89.6 | USB1.SHIELD5 7,89.6 | USB1.SHIELD5 5.62,88.82 | USB1.SHIELD5 | 5.61,90.47 USB1.SHIELD5 | USB1.SHIELD2 5.61,80.21 | USB1.SHIELD2 6.71,80.97 | USB1.SHIELD2 4.08,80.97 | USB1.SHIELD4 1.43,81.86 | USB1.SHIELD4 2.57,80.97 | USB1.SHIELD4 0.56,80.97
  other vias: 14.84,80.96 16.31,84.38 21.31,86.44 24.41,80.8 33.54,86.64 27.89,91.33 10.48,85.01 4.48,79.89 3.37,87.35 3.33,85.29 41,90.37 30.72,79.38 35.6,92.15 35.04,81.99 27.02,88.71 7.41,89.43 8.24,86.85 13.05,86.77 14.67,86.17 3.84,81.93 1.42,87.25 1.34,83.32 45,13 64,38 53,35.5 10.5,3 45.5,3 80.5,3 26.67,96.04 52.39,77.95 51.12,77.95 69.37,59.05 95.57,87.15 96.68,89.06 93.66,70.8 92.08,70.17 92.55,54.61
  pour Top: -0.5,100.5 -0.5,-0.5 100.5,-0.5 100.5,100.5
  pour Bottom: 100.5,100.5 100.5,-0.5 -0.5,-0.5 -0.5,100.5
GRID1  (via drill 0.35)
  Top 0.305: v31.99,68.42 31.99,70.24 | 31.99,70.24 SEG1.8 | v31.99,53.5 32,53.49 SEG1.3 | U1.2 v55.09,92.08 | v55.09,72.07 32.07,72.07 31.99,71.99 31.99,70.24
  Bottom 0.305: v31.99,53.5 v31.99,68.42 | v55.09,92.08 v55.09,72.07
GRID2  (via drill 0.35)  (1 unrouted)
  Top 0.305: U1.11 72.71,80.64 72.55,80.64 v68.1,80.64 | v68.1,73.18 68,73.08 SEG9.8
  Bottom 0.305: v68.1,80.64 v68.1,73.18
GRID3  (via drill 0.35, 0.35 pad 0.55)
  Top 0.305: v8.03,32.86 8,32.89 SEG3.8 8,39.24 v8.13,39.37 | v8.03,22.86 8.03,18.78 SEG3.3 | U1.6 v43.66,87 | v43.66,55.56 43.22,55.12 v8.13,55.12
  Bottom 0.305: v8.03,32.86 v8.03,22.86 | v43.66,87 v43.66,55.56 | v8.13,55.12 v8.13,39.37
GRID4  (via drill 0.35, 0.35 pad 0.55)
  Top 0.305: v22.08,35.24 v22.08,35.25 22.08,37.17 SEG4.8 22,39.3 v22.07,39.37 | v22,22.86 SEG4.3 | U1.7 v45.09,85.72 | v44.77,54.29 v22.23,54.29
  Bottom 0.305: v22.08,35.24 22.08,22.94 v22,22.86 | v45.09,85.72 44.77,85.41 v44.77,54.29 | v22.23,54.29 22.23,39.53 v22.07,39.37
GRID5  (via drill 0.35, 0.35 pad 0.55)
  Top 0.305: v43.18,35.24 43.18,37.07 SEG5.8 43,39.35 v43.02,39.37 | v43.02,22.86 43.02,18.77 SEG5.3 | U1.3 v58.58,90.81 | v58.58,48.9 v43.18,48.9
  Bottom 0.305: v43.18,35.24 43.18,23.02 v43.02,22.86 | v58.58,90.81 v58.58,48.9 | v43.18,48.9 43.02,48.74 v43.02,39.37
GRID6  (via drill 0.35, 0.35 pad 0.55)
  Top 0.305: SEG6.8 | 56.67,36.92 56.87,37.12 SEG6.8 | U1.10 v57.15,81.92 | v56.99,20.8 57,20.79 SEG6.3 | v56.99,39.37 SEG6.8
  Bottom 0.305: v57.15,81.92 56.99,81.76 v56.99,39.37 v56.99,20.8
GRID7  (via drill 0.35, 0.35 pad 0.55)
  Top 0.305: v78.25,35.24 78.25,37 SEG7.8 78,39.32 v77.95,39.37 | v78.33,22.86 78.33,19.08 SEG7.3 | U1.5 v77.47,88.27
  Bottom 0.305: v78.25,35.24 78.25,22.94 v78.33,22.86 | v77.47,88.27 77.47,39.85 v77.95,39.37
GRID8  (via drill 0.35)
  Top 0.305: U1.8 v81.44,84.45 | v91.92,39.37 92,39.29 SEG8.8 SEG8.3 | v82.07,60.33 v91.92,60.33
  Bottom 0.305: v81.44,84.45 82.07,83.82 v82.07,60.33 | v91.92,60.33 v91.92,39.37
N$1
  Top 0.203: C8.1 12.19,81.84 11.87,82.15 IC5.4
N$2
  Top 0.203: C9.1 18.34,86.58 18.23,86.58 | 18.23,86.58 Q3.P$1 | IC5.7 15.68,86.17 16.1,86.58 18.23,86.58
N$3
  Top 0.203: C10.1 20.1,84.31 Q3.P$3 20.07,85.34 19.92,85.49 17.46,85.49 16.95,84.98 IC5.8
N$4
  Top 0.203: C15.2 15.32,81.24 15.08,81.47 15.08,84.45 14.61,84.93 12.22,84.93 11.87,85.28 IC5.13
N$5  (via drill 0.25)
  Top 0.203: IC5.5 13.14,84.01 12.88,84.27 9.66,84.27 v9.6,84.22 | R8.2 9.91,81.29 v9.6,81.6
  Bottom 0.203: v9.6,81.6 v9.6,84.22
N$8
  Top 0.203: IC5.6 14.41,84.25 14.06,84.6 11.75,84.6 11.25,85.1 11.25,89.79 R9.2
N$9  (via drill 0.45)
  Top 0.406: USB1.A4/B9 5.75,87.74 5.28,87.27 v4.63,87.27 3.49,88.42 3.49,90.49 2.82,91.16 L2.1 | USB1.B4/A9 5.75,82.84 5.32,83.27 v4.55,83.27
  Bottom 0.406: v4.55,83.27 4.55,87.19 v4.63,87.27
N$10
  Top 0.203: USB1.B5 5.74,83.54 4.95,84.33 3.21,84.33 2.87,83.99 2.87,80.02 2.24,79.39 R10.2
N$11
  Top 0.203: USB1.A5 3.11,86.54 2.54,85.97 2.54,80.25 2.3,80.01 1.27,80.01 0.87,79.61 R11.2
N$12
  Top 0.203: C24.1 34.56,87.19 Q4.P$1 34.14,88.69 34.14,89.21 32.56,90.79 30.58,90.79 30.43,90.64 29.56,90.64 IC6.7
N$13
  Top 0.203: IC6.8 28.83,91.04 30.29,91.04 30.37,91.13 32.71,91.13 33.02,91.44 33.37,91.44 33.84,90.97 33.84,90.89 Q4.P$3 34.49,91.44 34.92,91.44 35.91,90.46 C25.1
N$14  (via drill 0.35)
  Top 0.305: R13.2 v84.61,76.83 | v84.61,85.72 U1.18
  Bottom 0.305: v84.61,76.83 v84.61,85.72
N$131  (1 unrouted)
RESET  (via drill 0.25, 0.3)
  Top 0.203: v25.82,83.35 v25.83,83.34 30.1,83.34 IC6.29 31.51,81.93 31.51,80.29 | C15.1 18.41,81.24 18.79,81.61 v18.79,81.85 | 31.51,80.29 31.51,79.69 32.05,79.16 34.29,79.16 | R12.2 31.52,80.3 31.51,80.29 | 38.46,79.16 34.29,79.16 | ISP1.5 38.13,81.57 38.46,81.24 38.46,79.16 | U$2.RST 34.3,79.15 34.29,79.16 | U$2.RST1 34.97,92.91 35.12,92.76 35.12,91.95 35.88,91.19 41.69,91.19 42.03,90.84 42.03,79.33 41.85,79.16 38.46,79.16
  Bottom 0.203: v18.79,81.85 24.32,81.85 v25.82,83.35
SEG1  (via drill 0.35, 0.35 pad 0.55)
  Top 0.305: v2.09,41.27 10.65,41.27 | 80.49,41.27 v87.79,41.27 94.46,41.27 94.54,41.19 SEG8.7 94.76,37.47 | 80.49,41.27 v71.91,41.27 v59.69,41.27 v45.72,41.27 v35.24,41.27 v24.62,41.27 10.65,41.27 | 10.65,37.36 SEG3.7 10.54,41.16 10.65,41.27 | v24.62,39.37 24.62,37.33 SEG4.7 | v45.72,39.37 45.72,37.43 SEG5.7 | 59.69,37.4 SEG6.7 59.54,39.22 v59.69,39.37 | 80.79,37.5 SEG7.7 80.54,41.22 80.49,41.27 | U1.14 v90.17,80.64 | SEG9.7 v70.54,68.42 | SEG1.7 v34.54,68.42
  Bottom 0.305: v24.62,41.27 v24.62,39.37 | v45.72,41.27 v45.72,39.37 | v59.69,39.37 v59.69,41.27 | v90.17,80.64 90.17,63.82 87.79,61.44 v87.79,41.27 | v70.54,68.42 71.28,67.68 71.28,50.01 71.91,49.37 v71.91,41.27 | v34.54,68.42 35.24,67.72 v35.24,41.27
SEG2  (via drill 0.35, 0.35 pad 0.55)
  Top 0.305: v3.03,42.23 v13.19,42.23 v27.16,42.23 v37.47,42.23 v48.26,42.23 v62.23,42.23 v73.98,42.23 v83.33,42.23 v93.82,42.23 96.86,42.23 97.08,42.01 SEG8.6 97.3,37.47 | SEG3.6 13.19,37.36 v13.19,39.37 | SEG4.6 27.16,37.33 v27.16,39.37 | SEG5.6 48.26,37.43 v48.26,39.37 | 62.23,37.4 SEG6.6 62.08,39.22 v62.23,39.37 | 83.33,37.5 SEG7.6 83.08,39.12 v83.33,39.37 | U1.16 v91.44,83.19 | v93.82,61.75 v91.44,61.75 | SEG9.6 v73.08,68.42 | SEG1.6 v37.08,68.42
  Bottom 0.305: v13.19,39.37 v13.19,42.23 | v27.16,39.37 v27.16,42.23 | v48.26,39.37 v48.26,42.23 | v62.23,42.23 v62.23,39.37 | v83.33,39.37 v83.33,42.23 | v93.82,42.23 v93.82,61.75 | v91.44,61.75 v91.44,83.19 | v73.08,68.42 73.82,67.68 73.82,42.39 v73.98,42.23 | v37.08,68.42 37.47,68.04 v37.47,42.23
SEG3  (via drill 0.35, 0.35 pad 0.55)
  Top 0.305: v3.33,43.18 v9.06,43.18 v23.04,43.18 v34.13,43.18 v44.13,43.18 v58.1,43.18 v70.64,43.18 v79.2,43.18 v93.17,43.18 | SEG3.4 10.54,20.75 v10.34,20.95 | v24.62,20.95 24.62,18.83 SEG4.4 | SEG5.4 45.4,18.89 v45.4,20.95 | SEG6.4 59.37,18.92 v59.37,20.8 | SEG7.4 80.54,20.89 v80.47,20.95 | SEG8.4 94.54,20.86 v94.44,20.95 | U1.20 v92.71,88.27 | SEG9.4 v70.54,49.85 | SEG1.4 v34.54,49.85
  Bottom 0.305: v10.34,20.95 9.06,22.23 v9.06,43.18 | v24.62,20.95 23.04,22.54 v23.04,43.18 | v45.4,20.95 44.13,22.23 v44.13,43.18 | v59.37,20.8 58.1,22.07 v58.1,43.18 | v80.47,20.95 79.2,22.23 v79.2,43.18 | v94.44,20.95 93.17,22.23 v93.17,43.18 93.17,62.09 92.71,62.55 v92.71,88.27 | v70.64,43.18 70.54,43.28 v70.54,49.85 | v34.54,49.85 34.54,43.59 v34.13,43.18
SEG4  (via drill 0.35, 0.35 pad 0.55)
  Top 0.305: v3.33,44.13 v6.84,44.13 v17.95,44.13 v28.57,44.13 v41.59,44.13 v55.56,44.13 v65.72,44.13 v76.66,44.13 v90.63,44.13 v97.79,44.13 | SEG3.2 5.46,22.75 v5.57,22.86 | SEG4.2 19.46,22.62 v19.23,22.86 | SEG5.2 40.46,22.68 v40.64,22.86 | SEG6.2 54.46,22.71 v54.61,22.86 | SEG7.2 75.46,20.25 v75.07,20.64 | SEG8.2 89.46,22.76 v89.36,22.86 | U1.23 v94.61,92.08 | SEG9.2 v65.46,49.85 | SEG1.2 v29.46,49.85
  Bottom 0.305: v6.84,44.13 6.84,24.13 v5.57,22.86 | v19.23,22.86 17.95,24.13 v17.95,44.13 | v40.64,22.86 41.59,23.81 v41.59,44.13 | v55.56,44.13 55.56,23.81 v54.61,22.86 | v75.07,20.64 76.66,22.23 v76.66,44.13 | v90.63,44.13 90.63,24.13 v89.36,22.86 | v94.61,92.08 97.79,88.9 v97.79,44.13 | v65.46,49.85 65.46,44.4 v65.72,44.13 | v29.46,49.85 28.57,48.96 v28.57,44.13
SEG5  (via drill 0.35, 0.35 pad 0.55)
  Top 0.305: v3.97,45.09 v14.46,45.09 v27.15,45.09 v36.2,45.09 v50.48,45.09 v63.18,45.09 v71.26,45.09 v85.23,45.09 v96.68,45.09 | v3.03,21.27 2.92,21.16 SEG3.1 | SEG4.1 16.92,20.72 v16.68,20.95 | SEG5.1 37.92,20.5 v37.47,20.95 | SEG6.1 51.92,20.79 v51.75,20.95 | SEG7.1 72.92,20.57 v72.53,20.95 | SEG8.1 86.92,20.54 v86.5,20.95 | U1.22 v93.98,90.81 | SEG9.1 v62.92,49.85 | SEG1.1 v26.92,49.85
  Bottom 0.305: v3.03,21.27 1.76,22.54 1.76,40.01 3.97,42.21 v3.97,45.09 | v16.68,20.95 16.68,33.97 14.46,36.2 v14.46,45.09 | v37.47,20.95 36.2,22.23 v36.2,45.09 | v51.75,20.95 50.48,22.23 v50.48,45.09 | v72.53,20.95 71.26,22.23 v71.26,45.09 | v86.5,20.95 85.23,22.23 v85.23,45.09 | v93.98,90.81 96.68,88.11 v96.68,45.09 | v62.92,49.85 62.92,45.35 v63.18,45.09 | v26.92,49.85 26.92,45.31 v27.15,45.09
SEG6  (via drill 0.35, 0.35 pad 0.55)
  Top 0.305: v4.6,46.04 v5.89,46.04 v18.91,46.04 v30.16,46.04 v40.64,46.04 v54.61,46.04 v66.2,46.04 v75.71,46.04 v89.68,46.04 v94.46,46.04 | 5.57,37.36 SEG3.9 5.46,39.26 v5.57,39.37 | SEG4.9 19.46,39.32 v19.32,39.46 | SEG5.9 40.64,37.43 v40.64,39.37 | SEG6.9 54.61,37.4 v54.61,39.37 | SEG7.9 75.71,37.5 v75.71,39.37 | 89.68,37.47 SEG8.9 89.46,39.15 v89.68,39.37 | U1.21 v93.34,89.53 | SEG9.9 v65.46,68.42 | SEG1.9 v29.46,68.42
  Bottom 0.305: v5.89,46.04 5.89,39.69 v5.57,39.37 | v19.32,39.46 18.91,39.87 v18.91,46.04 | v40.64,39.37 v40.64,46.04 | v54.61,39.37 v54.61,46.04 | v75.71,39.37 v75.71,46.04 | v89.68,39.37 v89.68,46.04 | v93.34,89.53 94.46,88.42 v94.46,46.04 | v65.46,68.42 66.2,67.68 v66.2,46.04 | v29.46,68.42 30.16,67.72 v30.16,46.04
SEG7  (via drill 0.35, 0.35 pad 0.55)
  Top 0.305: v5.25,46.99 v17,46.99 v27.62,46.99 v38.1,46.99 v52.07,46.99 v63.66,46.99 v73.17,46.99 v87.14,46.99 v90.81,46.99 | 3.12,37.45 SEG3.10 2.92,39.17 v3.12,39.37 | SEG4.10 17,37.33 v17,39.37 | SEG5.10 38.1,37.43 v38.1,39.37 | SEG6.10 52.07,37.4 v52.07,39.37 | SEG7.10 73.17,37.5 v73.17,39.37 | 87.14,37.47 SEG8.10 86.92,39.15 v87.14,39.37 | U1.15 v90.81,81.92 | SEG9.10 v62.92,68.42 | SEG1.10 v26.92,68.42
  Bottom 0.305: v3.12,39.37 5.25,41.5 v5.25,46.99 | v17,39.37 v17,46.99 | v38.1,39.37 v38.1,46.99 | v52.07,39.37 v52.07,46.99 | v73.17,39.37 v73.17,46.99 | v87.14,39.37 v87.14,46.99 | v90.81,46.99 v90.81,81.92 | v62.92,68.42 63.66,67.68 v63.66,46.99 | v26.92,68.42 27.62,67.72 v27.62,46.99
SEG8  (via drill 0.35, 0.35 pad 0.55)
  Top 0.305: v6.05,47.94 v11.92,47.94 v25.89,47.94 v36.83,47.94 v46.99,47.94 v60.96,47.94 73.18,47.94 | 73.18,47.94 v82.06,47.94 v96.03,47.94 | SEG3.5 13.08,22.34 v11.92,23.5 | SEG5.5 48.08,22.41 v46.99,23.5 | SEG4.5 27.08,22.31 v25.89,23.5 | SEG6.5 62.08,20.79 v62.07,20.8 | SEG7.5 83.08,22.47 v82.06,23.5 | SEG8.5 97.08,22.44 v96.03,23.5 | U1.17 v95.25,84.45 | 73.18,47.94 73.08,48.05 SEG9.5 | SEG1.5 37.08,50.1 v36.83,49.85
  Bottom 0.305: v11.92,23.5 v11.92,47.94 | v46.99,23.5 v46.99,47.94 | v25.89,23.5 v25.89,47.94 | v60.96,47.94 60.96,21.91 v62.07,20.8 | v82.06,23.5 v82.06,47.94 | v96.03,23.5 v96.03,47.94 96.03,83.68 v95.25,84.45 | v36.83,49.85 v36.83,47.94

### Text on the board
Top: Multiplication trainer 1.0
tPlace: D12 | D11 | D10 | D9 | D8 | D7 | D6 | D5 | D4 | D3 | D2 | GND | RST | D0 | D1 | D13 | +3V3 | AREF | A0 | A1 | A2 | A3 | A4 | A5 | A6 | A7 | +5V | RST | GND | VIN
